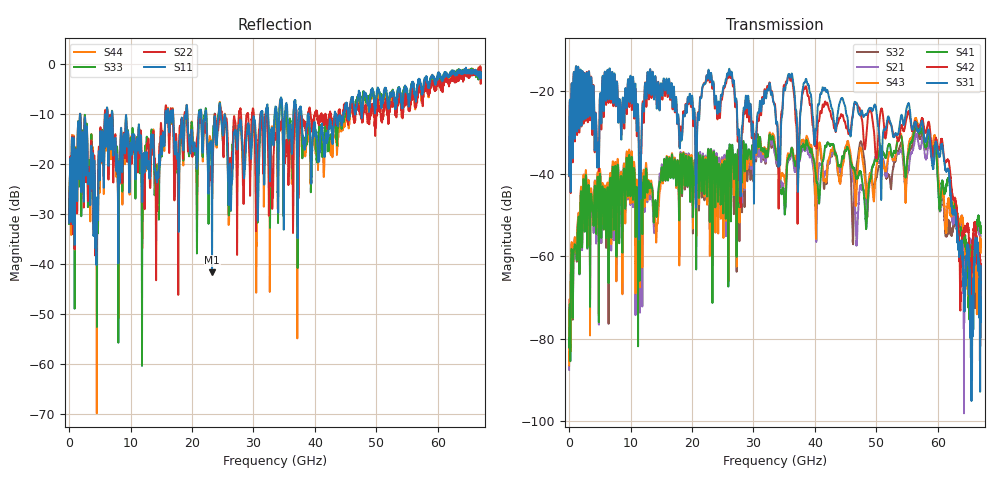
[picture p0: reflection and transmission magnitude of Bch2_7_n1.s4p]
!Agilent Technologies,N5247A,US51170199,A.09.90.13
!Agilent N5247A: A.09.90.13
!Date: Wednesday, October 17, 2018 17:38:19
!Correction: S11(Full 4 Port(1,2,3,4))
!S12(Full 4 Port(1,2,3,4))
!S13(Full 4 Port(1,2,3,4))
!S14(Full 4 Port(1,2,3,4))
!S21(Full 4 Port(1,2,3,4))
!S22(Full 4 Port(1,2,3,4))
!S23(Full 4 Port(1,2,3,4))
!S24(Full 4 Port(1,2,3,4))
!S31(Full 4 Port(1,2,3,4))
!S32(Full 4 Port(1,2,3,4))
!S33(Full 4 Port(1,2,3,4))
!S34(Full 4 Port(1,2,3,4))
!S41(Full 4 Port(1,2,3,4))
!S42(Full 4 Port(1,2,3,4))
!S43(Full 4 Port(1,2,3,4))
!S44(Full 4 Port(1,2,3,4))
!S4P File: Measurements: <S11,S12,S13,S14>,
!<S21,S22,S23,S24>,
!<S31,S32,S33,S34>,
!<S41,S42,S43,S44>:
# Hz S  dB  R 50
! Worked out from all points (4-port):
!   6701 points, 10 MHz to 67 GHz, reference 50 ohm
!   strongest paths, dB at 10 MHz, 16.76 GHz, 33.51 GHz, 50.25 GHz, 67 GHz:
!     S31: -40.5, -20.5, -24.0, -28.1, -62.5
!     S42: -40.7, -21.2, -23.3, -32.2, -65.8
!     S41: -79.9, -35.4, -33.5, -36.2, -53.9
!     S43: -86.5, -35.1, -32.8, -36.2, -59.2
!     S21: -87.6, -35.6, -35.0, -37.4, -53.9
!     S32: -85.3, -35.4, -35.2, -39.3, -68.1
!   lowest |S11| = -41.6 dB at 23.27 GHz (marker M1), VSWR 1.02, Z = 49.6 - j0.714 ohm
!   |S11| at or under -10 dB: 7.046 GHz to 15.67 GHz (8.627 GHz wide, 75.9 % of centre); 24.66 GHz to 31.16 GHz (6.499 GHz wide, 23.3 % of centre); 38.96 GHz to 43.22 GHz (4.259 GHz wide, 10.4 % of centre)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
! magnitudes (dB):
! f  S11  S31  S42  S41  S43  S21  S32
! 10 MHz  -31.7  -40.5  -40.7  -79.9  -86.5  -87.6  -85.3
! 2.54 GHz  -11.1  -15.8  -15.8  -53.9  -53.2  -53.4  -53.0
! 23.27 GHz  -41.6  -18.2  -19.0  -40.9  -39.2  -40.4  -41.5
! 48.33 GHz  -6.3  -25.7  -31.5  -53.3  -45.0  -47.8  -43.5
! 56.55 GHz  -5.7  -29.0  -28.2  -27.8  -27.0  -30.6  -29.0
! 64.42 GHz  -1.7  -64.5  -53.1  -55.8  -56.5  -67.0  -60.3
! 67 GHz  -2.8  -62.5  -65.8  -53.9  -59.2  -53.9  -68.1
